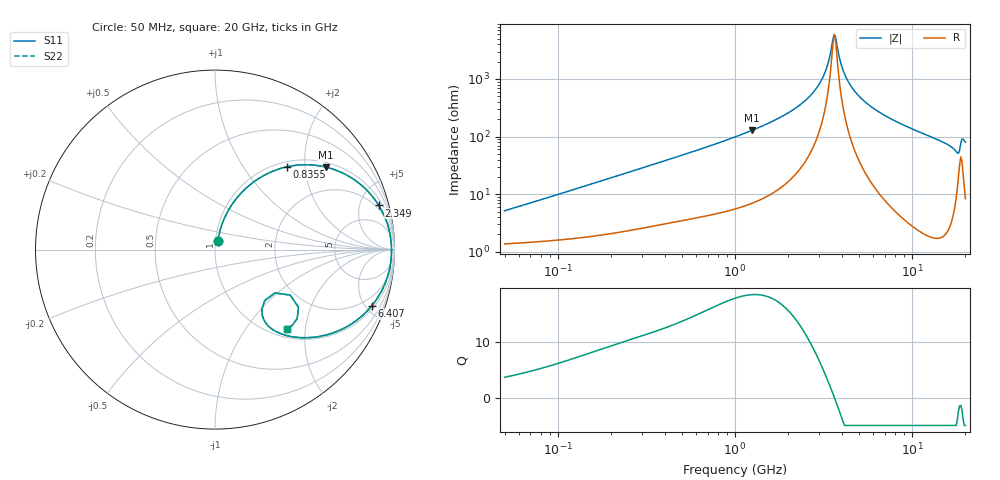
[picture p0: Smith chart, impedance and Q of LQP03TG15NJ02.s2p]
!Murata Part Number: LQP03TG15NJ02
!These Parameters are Measured in Series Mode Connection
!  o--[Z]--o
!Port1  Port2
!  o-------o
!Freq. Start=50[MHz] Stop=20[GHz], 401[Steps]
# Hz S RI R 50
!Freq.(Hz) S11(Real) S11(Imag) S21(Real) S21(Imag) S12(Real) S12(Imag) S22(Real) S22(Imag)
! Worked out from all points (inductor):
!   401 points, 50 MHz to 20 GHz, reference 50 ohm
!   read as one part in series: L = 15.7 nH near 51.52 MHz
!   highest Q = 18.5 at 1.252 GHz (marker M1), where L = 16.4 nH
!   self-resonance near 3.626 GHz
!   S11 on the Smith chart (normalised r, x): 50 MHz: 1.03, +0.10; 835.5 MHz: 1.10, +1.61; 2.349 GHz: 1.57, +7.23; 6.407 GHz: 1.22, -5.50; 20 GHz: 1.17, -1.59
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5e7  0.0159 0.0483  0.9841 -0.0483  0.9841 -0.0483  0.0159 0.0483
1.364002e8  0.0336 0.1255  0.9664 -0.1255  0.9664 -0.1255  0.0336 0.1255
3.721004e8  0.1301 0.2976  0.8699 -0.2976  0.8699 -0.2976  0.1301 0.2976
8.354841e8  0.4001 0.4611  0.5999 -0.4611  0.5999 -0.4611  0.4001 0.4611
1e9  0.4933 0.4727  0.5067 -0.4727  0.5067 -0.4727  0.4933 0.4727
1.251922e9  0.6183 0.4595  0.3817 -0.4595  0.3817 -0.4595  0.6183 0.4595
1.793498e9  0.8071 0.3661  0.1929 -0.3661  0.1929 -0.3661  0.8071 0.3661
2.348516e9  0.9127 0.2457  0.0873 -0.2457  0.0873 -0.2457  0.9127 0.2457
2.728004e9  0.9519 0.1663  0.0481 -0.1663  0.0481 -0.1663  0.9519 0.1663
3.216634e9  0.9773 0.0728  0.0227 -0.0728  0.0227 -0.0728  0.9773 0.0728
3.626126e9  0.9836 0.00271  0.0164 -0.00271  0.0164 -0.00271  0.9836 0.00271
3.736399e9  0.9836 -0.0149  0.0164 0.0149  0.0164 0.0149  0.9836 -0.0149
4.087748e9  0.9797 -0.0678  0.0203 0.0678  0.0203 0.0678  0.9797 -0.0678
4.472136e9  0.9699 -0.1201  0.0301 0.1201  0.0301 0.1201  0.9699 -0.1201
5.194772e9  0.9408 -0.2047  0.0592 0.2047  0.0592 0.2047  0.9408 -0.2047
6.406762e9  0.8737 -0.3129  0.1263 0.3129  0.1263 0.3129  0.8737 -0.3129
7.442007e9  0.8084 -0.3787  0.1916 0.3787  0.1916 0.3787  0.8084 -0.3787
1.257102e10  0.505 -0.491  0.495 0.491  0.495 0.491  0.505 -0.491
1.573793e10  0.3571 -0.4646  0.6429 0.4646  0.6429 0.4646  0.3571 -0.4646
1.747767e10  0.2739 -0.3948  0.7261 0.3948  0.7261 0.3948  0.2739 -0.3948
1.855685e10  0.3338 -0.2417  0.6662 0.2417  0.6662 0.2417  0.3338 -0.2417
2e10  0.4013 -0.4406  0.5987 0.4406  0.5987 0.4406  0.4013 -0.4406
